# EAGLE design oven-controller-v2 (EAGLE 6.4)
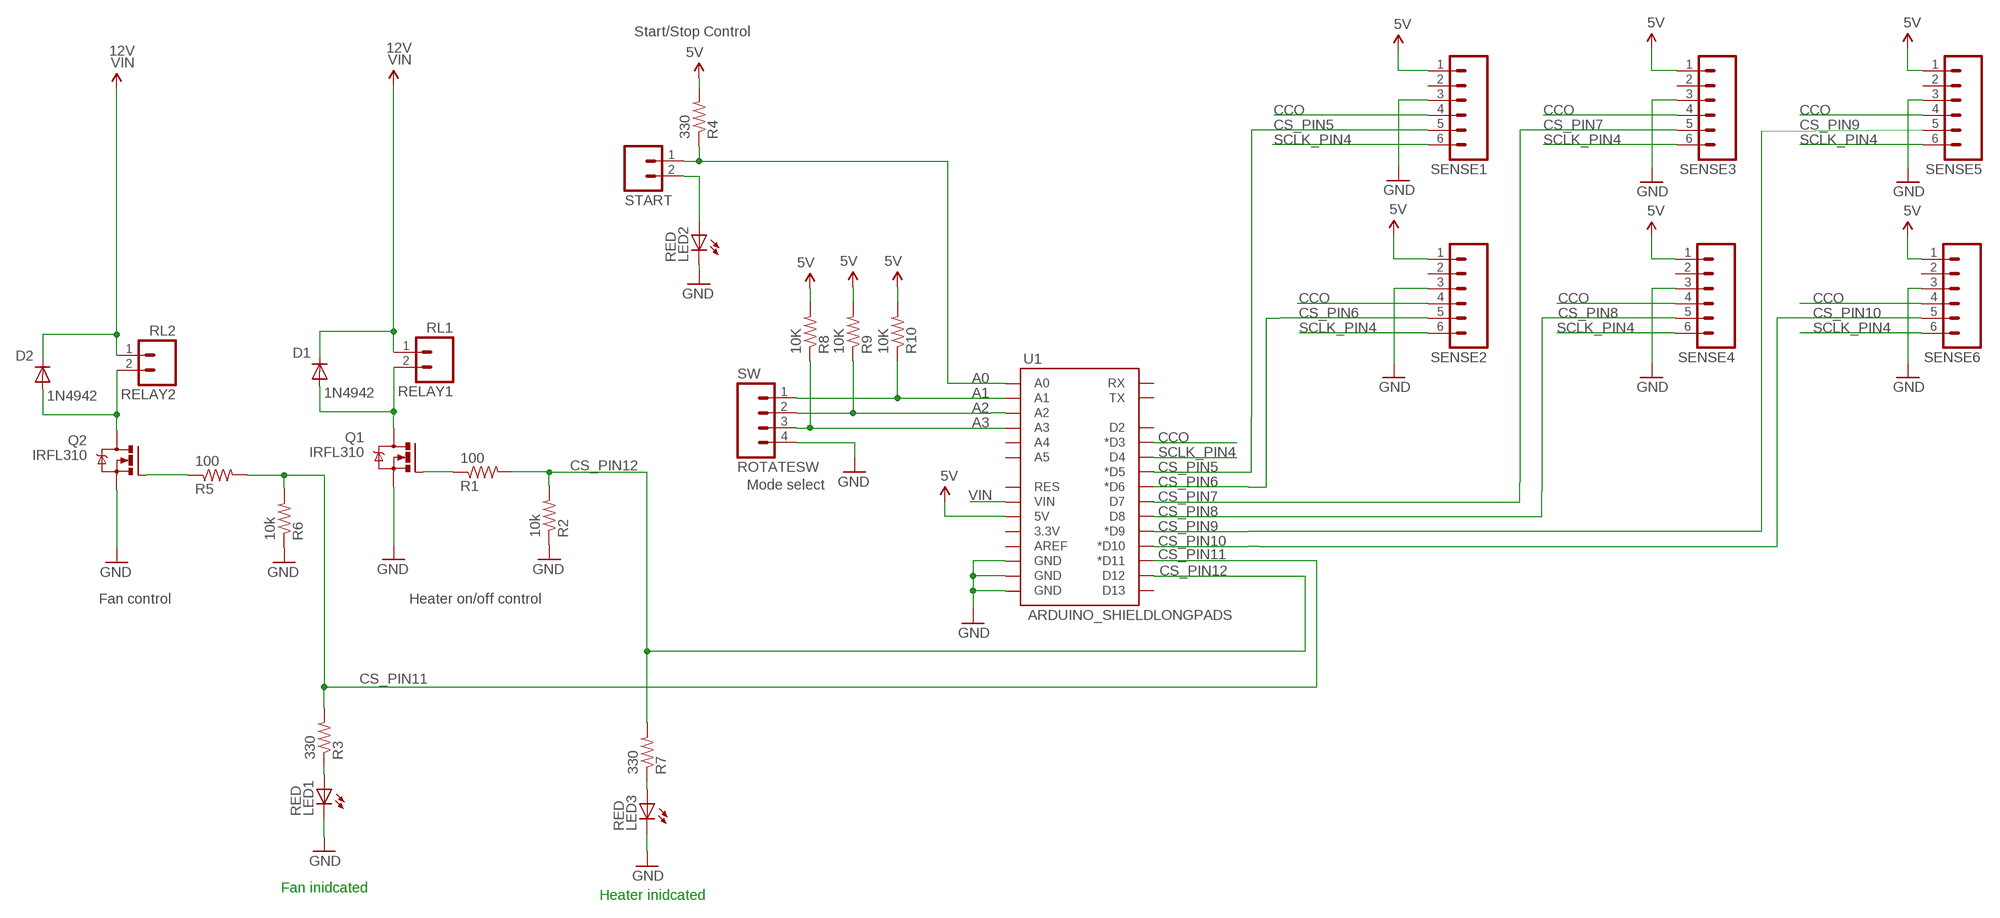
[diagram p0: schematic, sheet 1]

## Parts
D1  1N4942  [DO41-10]
D2  1N4942  [DO41-10]
LED1  RED  LED5MM  [LED5MM]
LED2  RED  LED5MM  [LED5MM]
LED3  RED  LED5MM  [LED5MM]
Q1  IRFL310  IRF520  [TO220BV]
Q2  IRFL310  IRF520  [TO220BV]
R1  100  RESISTORAXIAL-0.3  [AXIAL-0.3]
R2  10k  RESISTORAXIAL-0.3  [AXIAL-0.3]
R3  330  RESISTORAXIAL-0.3  [AXIAL-0.3]
R4  330  RESISTORAXIAL-0.3  [AXIAL-0.3]
R5  100  RESISTORAXIAL-0.3  [AXIAL-0.3]
R6  10k  RESISTORAXIAL-0.3  [AXIAL-0.3]
R7  330  RESISTORAXIAL-0.3  [AXIAL-0.3]
R8  10K  RESISTORAXIAL-0.3  [AXIAL-0.3]
R9  10K  RESISTORAXIAL-0.3  [AXIAL-0.3]
R10  10K  RESISTORAXIAL-0.3  [AXIAL-0.3]
RELAY1  RL1  M023.5MM_LOCK  [SCREWTERMINAL-3.5MM-2_LOCK]
RELAY2  RL2  M023.5MM_LOCK  [SCREWTERMINAL-3.5MM-2_LOCK]
ROTATESW  SW  M04LOCK_LONGPADS  [1X04_LOCK_LONGPADS]
SENSE1  M06LOCK_LONGPADS  [1X06_LOCK_LONGPADS]
SENSE2  M06LOCK_LONGPADS  [1X06_LOCK_LONGPADS]
SENSE3  M06LOCK_LONGPADS  [1X06_LOCK_LONGPADS]
SENSE4  M06LOCK_LONGPADS  [1X06_LOCK_LONGPADS]
SENSE5  M06LOCK_LONGPADS  [1X06_LOCK_LONGPADS]
SENSE6  M06LOCK_LONGPADS  [1X06_LOCK_LONGPADS]
START  M023.5MM_LOCK  [SCREWTERMINAL-3.5MM-2_LOCK]
U1  ARDUINO_SHIELDLONGPADS  [DUEMILANOVE_SHIELD_LONGPADS]

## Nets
5V: R4.P$2 R8.P$2 R9.P$2 R10.P$2 SENSE1.1 SENSE2.1 SENSE3.1 SENSE4.1 SENSE5.1 SENSE6.1 U1.5V
A0: R4.P$1 START.1 U1.A0
A1: R10.P$1 ROTATESW.1 U1.A1
A2: R9.P$1 ROTATESW.2 U1.A2
A3: R8.P$1 ROTATESW.3 U1.A3
CCO: SENSE1.4 SENSE2.4 SENSE3.4 SENSE4.4 SENSE5.4 SENSE6.4 U1.D3(*D3)
CS_PIN5: SENSE1.5 U1.D5(*D5)
CS_PIN6: SENSE2.5 U1.D6(*D6)
CS_PIN7: SENSE3.5 U1.D7
CS_PIN8: SENSE4.5 U1.D8
CS_PIN9: SENSE5.5 U1.D9(*D9)
CS_PIN10: SENSE6.5 U1.D10(*D10)
CS_PIN11: R3.P$2 R5.P$2 R6.P$2 U1.D11(*D11)
CS_PIN12: R1.P$2 R2.P$2 R7.P$2 U1.D12
GND: LED1.K(C) LED2.K(C) LED3.K(C) Q1.S Q2.S R2.P$1 R6.P$1 ROTATESW.4 SENSE1.3 SENSE2.3 SENSE3.3 SENSE4.3 SENSE5.3 SENSE6.3 U1.GND@0(GND) U1.GND@1(GND) U1.GND@2(GND)
N$1: Q2.G R5.P$1
N$2: Q1.G R1.P$1
N$3: D1.A Q1.D RELAY1.2
N$4: D2.A Q2.D RELAY2.2
N$7: LED1.A R3.P$1
N$9: LED3.A R7.P$1
N$10: LED2.A START.2
SCLK_PIN4: SENSE1.6 SENSE2.6 SENSE3.6 SENSE4.6 SENSE5.6 SENSE6.6 U1.D4
VIN: D1.C D2.C RELAY1.1 RELAY2.1 U1.VIN
Unconnected: SENSE1.2 SENSE2.2 SENSE3.2 SENSE4.2 SENSE5.2 SENSE6.2 U1.3.3V U1.A4 U1.A5 U1.AREF U1.D2 U1.D13 U1.RES U1.RX U1.TX

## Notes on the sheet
- Start/Stop Control
- 12V | 12V
- Mode select
- Fan control | Heater on/off control
- Fan inidcated
- Heater inidcated

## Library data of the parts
D1 D2 = diode:1N4942: DIODE
LED1-LED3 = led:LED: LED
Q1 Q2 = transistor-power:IRF520: HEXFET Power MOSFET
R1-R10 = SparkFun-Passives:RESISTOR: Resistor
RELAY1 RELAY2 START = SparkFun-Connectors:M02: Header 2
ROTATESW = SparkFun-Connectors:M04: Header 4 Standard 4-pin 0.1" header. Use with straight break away headers (SKU : PRT-00116), right angle break away headers (PRT-00553), swiss pins (PRT-00743), machine pins (PRT-00117), and female headers (PRT-00115). Molex polarized connector foot print use with SKU : PRT-08231 with associated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
SENSE1-SENSE6 = SparkFun-Connectors:M06: Header 6 Standard 6-pin 0.1" header. Use with straight break away headers (SKU : PRT-00116), right angle break away headers (PRT-00553), swiss pins (PRT-00743), machine pins (PRT-00117), and female headers (PRT-00115). Molex polarized connector foot print use with SKU : PRT-08094 with associated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
U1 = SparkFun-Boards:ARDUINO_SHIELD: Arduino shield footprint

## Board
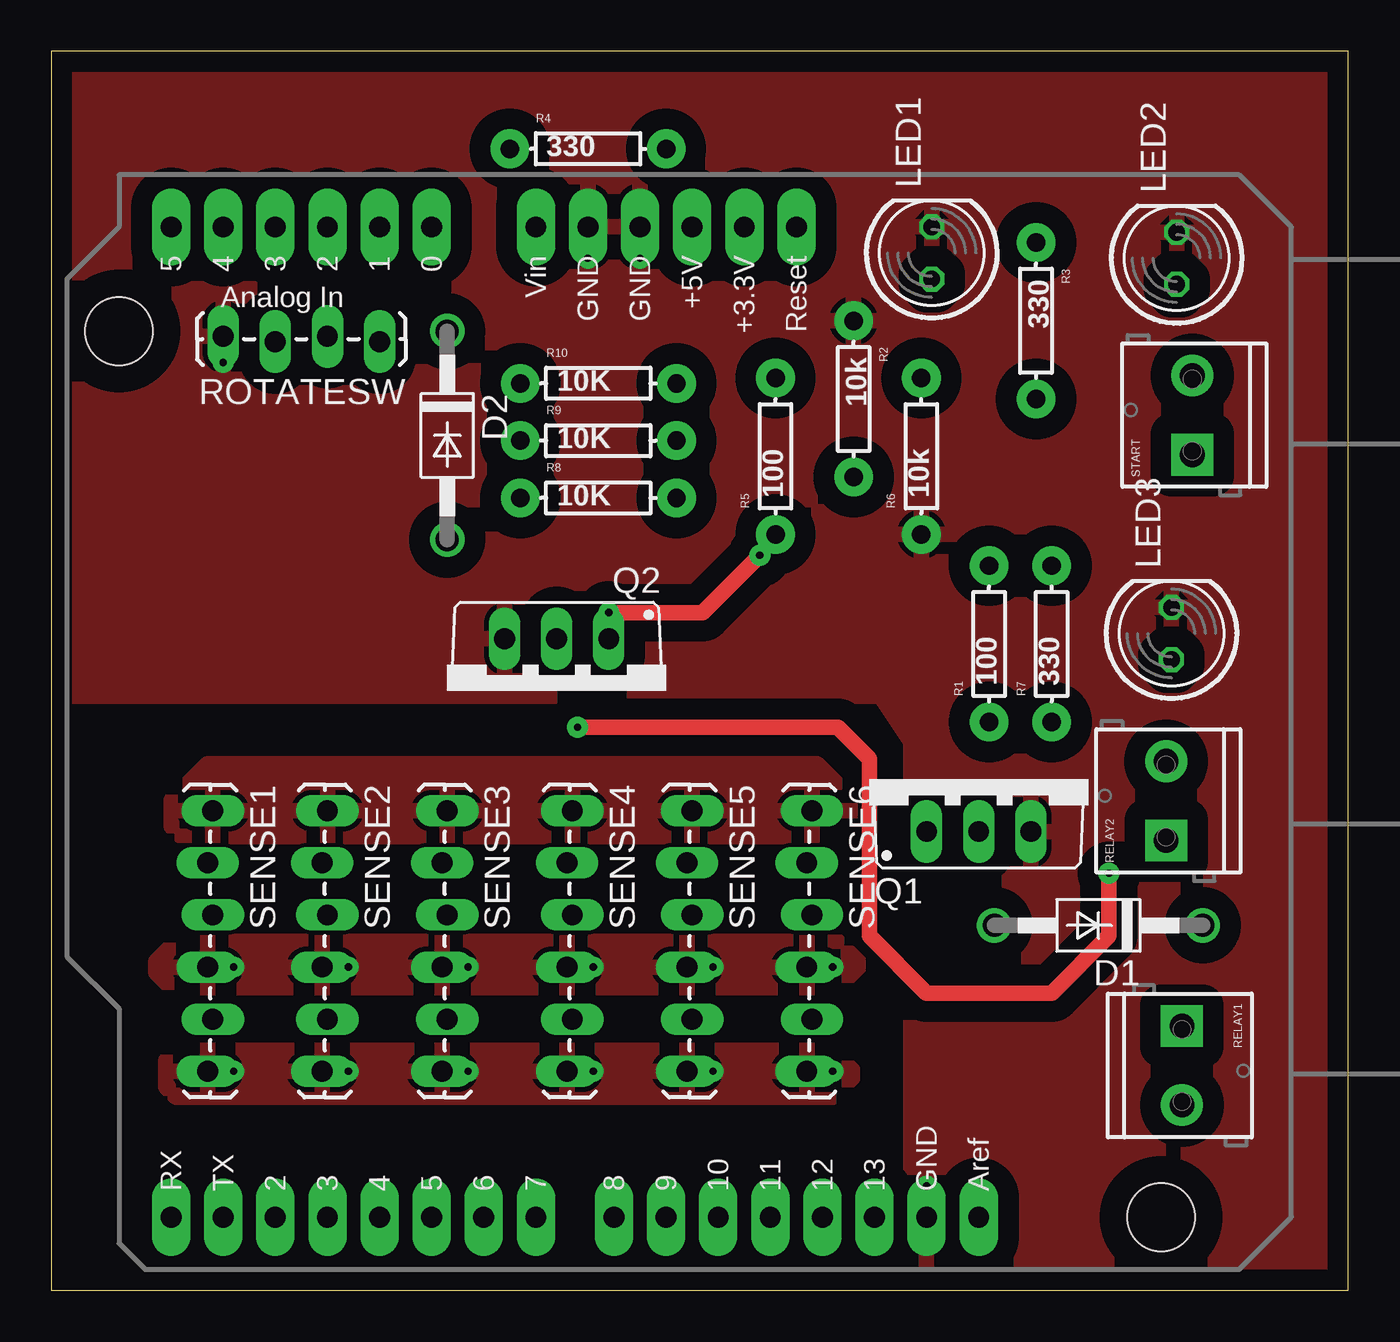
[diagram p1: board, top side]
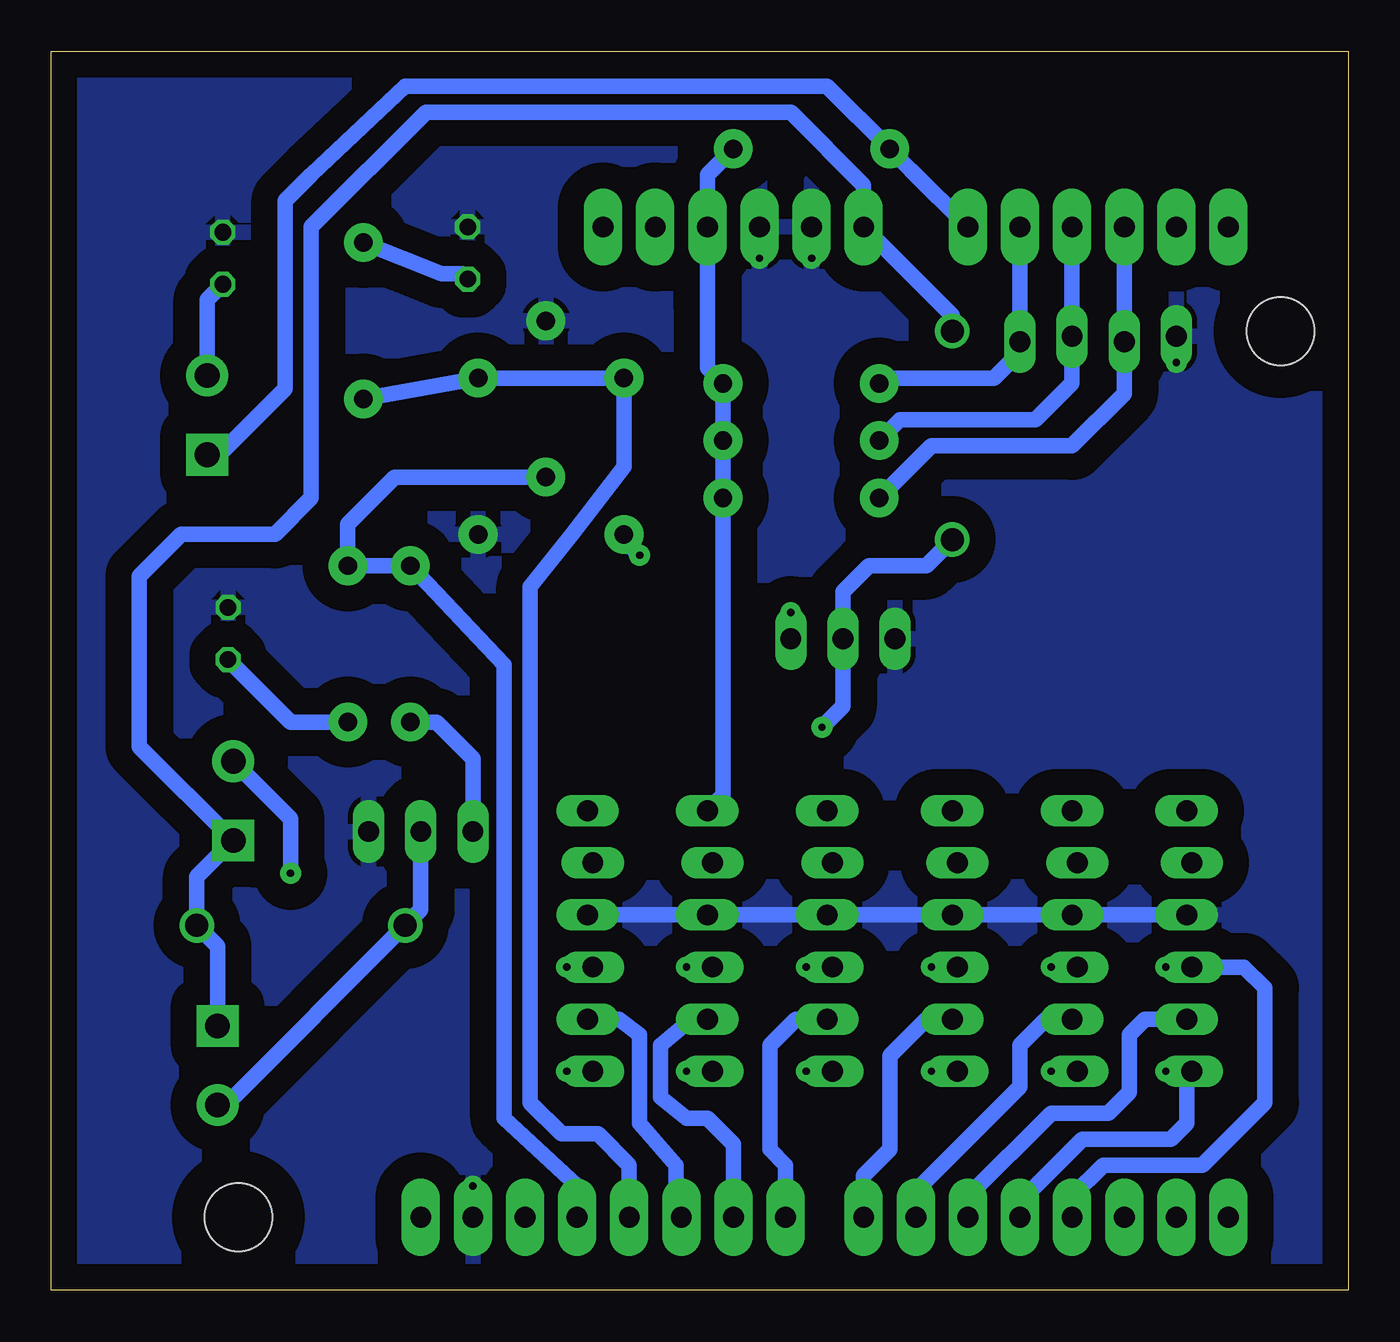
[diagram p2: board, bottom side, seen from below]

Size 63.23 x 60.38 mm. Coordinates in mm from the lower left corner, seen from the top.
Outline: 0,0 63.23,0 63.23,60.38 0,60.38 0,0
Copper layers (1*16): Top 0.0178mm / dielectric 59mil / Bottom 0.0178mm
Design rules "epl-lpkf": minimum track width 8mil, minimum drill 0.35mm, track to track 8mil, track to pad 8mil, pad to pad 8mil, via to via 8mil, smd to smd 8mil, copper to edge 15mil, drill to drill 15mil, minimum pad ring 8mil, minimum via ring 8mil, stop-mask expansion 3mil, vias tented up to drill 0mil, thermal gap 10mil

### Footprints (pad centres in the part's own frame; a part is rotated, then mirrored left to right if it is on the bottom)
DO41-10 = drill 1.118: A 5.08,0; C -5.08,0
LED5MM = drill 0.813 octagon: A -1.27,0; K 1.27,0
TO220BV = drill 1.016 long: D 0,-2.54; G -2.54,-2.54; S 2.54,-2.54
AXIAL-0.3 = drill 0.9 pad 1.88: P$1 -3.81,0; P$2 3.81,0
SCREWTERMINAL-3.5MM-2_LOCK = drill 1.2 pad 2.032 square: 1 -0.178,0 | drill 1.2 pad 2.032: 2 3.678,0
1X04_LOCK_LONGPADS = drill 1.016 long: 1 0,0; 2 2.54,-0.254; 3 5.08,0; 4 7.62,-0.254
1X06_LOCK_LONGPADS = drill 1.016 long: 1 0,0; 2 2.54,-0.254; 3 5.08,0; 4 7.62,-0.254; 5 10.16,0; 6 12.7,-0.254
DUEMILANOVE_SHIELD_LONGPADS = drill 1.016 pad 1.88 long: 3.3V 50.8,26.67; 5V 50.8,29.21; A0 50.8,41.91; A1 50.8,44.45; A2 50.8,46.99; A3 50.8,49.53; A4 50.8,52.07; A5 50.8,54.61; AREF 2.54,15.24; D2 2.54,49.53; D3 2.54,46.99; D4 2.54,44.45; D5 2.54,41.91; D6 2.54,39.37; D7 2.54,36.83; D8 2.54,33.02; D9 2.54,30.48; D10 2.54,27.94; D11 2.54,25.4; D12 2.54,22.86; D13 2.54,20.32; GND@0 50.8,31.75; GND@1 50.8,34.29; GND@2 2.54,17.78; RES 50.8,24.13; RX 2.54,54.61; TX 2.54,52.07; VIN 50.8,36.83 | hole 3.302: 45.72,57.15; 2.54,6.35

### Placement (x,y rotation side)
D1  51.05,17.78 180 top
D2  19.3,41.66 270 top
LED1  42.93,50.55 90 top
LED2  54.86,50.29 90 top
LED3  54.61,32 90 top
Q1  45.21,24.89 0 top
Q2  24.64,29.21 180 top
R1  45.72,31.5 90 top
R2  39.12,43.43 270 top
R3  48.01,47.24 270 top
R4  26.16,55.63 0 top
R5  35.31,40.64 90 top
R6  42.42,40.64 90 top
R7  48.77,31.5 90 top
R8  26.67,38.61 0 top
R9  26.67,41.4 0 top
R10  26.67,44.2 0 top
RELAY1  55.12,12.7 270 top
RELAY2  54.36,22.1 90 top
ROTATESW  16,46.23 180 top
SENSE1  7.87,23.37 270 top
SENSE2  13.46,23.37 270 top
SENSE3  19.3,23.37 270 top
SENSE4  25.4,23.37 270 top
SENSE5  31.24,23.37 270 top
SENSE6  37.08,23.37 270 top
START  55.63,40.89 90 top
U1  60.45,1.02 90 top

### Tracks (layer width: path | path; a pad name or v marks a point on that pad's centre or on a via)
5V
  Bottom 0.762: SENSE5.1 30.48,24.13 R8.P$2 R9.P$2 R10.P$2 31.24,44.96 31.24,48.01 U1.5V 31.24,54.36 R4.P$2
  pour Top: 5.84,23.88 6.6,24.64 7.62,25.65 37.34,25.65 39.12,23.88 39.12,23.11 38.1,22.1 6.35,22.1 5.84,22.61
A0
  Bottom 0.762: 18.54,51.56 U1.A0 21.34,54.61 R4.P$1 25.4,58.67 45.97,58.67 50.55,54.36 51.82,53.09 51.82,43.94 55.04,40.72 START.1
A1
  Bottom 0.762: U1.A1 ROTATESW.1 16,45.72 17.27,44.45 22.61,44.45 R10.P$1
A2
  Bottom 0.762: U1.A2 ROTATESW.2 13.46,44.2 15.24,42.42 21.84,42.42 R9.P$1
A3
  Bottom 0.762: U1.A3 ROTATESW.3 10.92,43.69 13.46,41.15 20.32,41.15 R8.P$1
CCO  (via drill 0.36 pad 1.02)
  Bottom 0.762: U1.D3 13.46,4.57 11.94,6.1 7.11,6.1 4.06,9.14 4.06,14.73 5.08,15.75 SENSE1.4
  other vias: 8.89,15.75 14.48,15.75 20.32,15.75 26.42,15.75 32.26,15.75 38.1,15.75
  pour Top: 6.6,16.76 5.84,16.76 5.08,16 5.08,15.49 5.84,14.73 38.35,14.73 39.37,15.75 39.37,16 38.35,17.02 6.86,17.02
CS_PIN5
  Bottom 0.762: SENSE1.5 9.91,13.21 10.67,12.45 10.67,9.65 11.43,8.89 11.68,8.64 14.48,8.64 18.54,4.57 U1.D5
CS_PIN6
  Bottom 0.762: SENSE2.5 14.73,13.21 16,11.94 16,9.91 20.83,5.08 21.08,4.83 U1.D6
CS_PIN7
  Bottom 0.762: SENSE3.5 20.57,13.21 22.35,11.43 22.35,6.86 23.62,5.59 U1.D7
CS_PIN8
  Bottom 0.762: SENSE4.5 26.92,13.21 28.19,11.94 28.19,6.86 27.43,6.1 U1.D8
CS_PIN9
  Bottom 0.762: SENSE5.5 32,13.21 33.53,11.94 33.53,9.4 32.26,8.38 31.24,8.38 29.97,7.11 U1.D9
CS_PIN10
  Bottom 0.762: SENSE6.5 35.56,13.21 34.54,12.45 34.54,8.13 32.77,6.1 32.77,3.81 U1.D10
CS_PIN11
  Bottom 0.762: R3.P$2 R6.P$2 R5.P$2 35.31,40.13 37.85,36.83 39.88,34.29 39.88,9.14 38.35,7.62 36.58,7.62 35.05,6.1 U1.D11
CS_PIN12
  Bottom 0.762: R2.P$2 46.48,39.62 48.77,37.34 R7.P$2 R1.P$2 41.15,30.48 41.15,8.38 37.59,5.08 U1.D12
GND  (via drill 0.36 pad 1.02)
  Bottom 0.762: SENSE1.3 SENSE2.3 SENSE3.3 SENSE4.3 SENSE5.3 SENSE6.3
  other vias: 28.7,50.29 26.16,50.29 8.38,45.21 42.67,5.08
  pour Bottom (isolate 1.27): -1.27,56.9 -1.27,-1.27 65.02,-1.27 64.52,61.47 -1.52,61.47
  pour Top (isolate 1.016): -1.52,61.72 -1.02,28.96 40.39,28.96 41.91,26.67 41.91,-0.25 65.02,-0.51 65.53,2.29 65.28,28.96 64.77,61.72
N$1  (via drill 0.36 pad 1.02)
  Top 0.762: v27.18,33.02 31.75,33.02 v34.54,35.81
  Bottom 0.762: Q2.G v27.18,33.02 | R5.P$1 35.31,36.58 v34.54,35.81
N$2
  Bottom 0.762: R1.P$1 44.45,27.69 42.67,25.91 Q1.G
N$3
  Bottom 0.762: RELAY1.2 54.73,9.02 D1.A 45.21,18.54 Q1.D
N$4  (via drill 0.36 pad 1.02)
  Top 0.762: v25.65,27.43 38.35,27.43 39.88,25.91 39.88,17.27 42.67,14.48 48.77,14.48 51.56,17.27 v51.56,20.32
  Bottom 0.762: D2.A 20.57,35.31 23.37,35.31 24.64,34.04 Q2.D 24.64,28.45 v25.65,27.43 | v51.56,20.32 51.56,22.98 RELAY2.2
N$7
  Bottom 0.762: R3.P$1 44.2,49.53 43.18,49.53 LED1.A
N$9
  Bottom 0.762: R7.P$1 51.56,27.69 LED3.A
N$10
  Bottom 0.762: START.2 55.63,48.26 LED2.A
SCLK_PIN4  (via drill 0.36 pad 1.02)
  Bottom 0.762: U1.D4 16,4.32 12.95,7.37 8.64,7.37 7.87,8.13 7.87,10.41 SENSE1.6
  other vias: 8.89,10.67 14.48,10.67 20.32,10.67 26.42,10.67 32.26,10.67 38.1,10.67
  pour Top: 38.35,11.43 39.12,10.67 39.12,10.41 38.1,9.4 6.1,9.4 5.59,9.91 5.59,11.18 6.1,11.68 37.85,11.68 38.35,11.18
VIN
  Bottom 0.762: RELAY1.1 55.12,16.76 D1.C 56.13,20.14 RELAY2.1 58.93,26.49 58.93,34.8 56.9,36.83 52.32,36.83 50.55,38.61 50.55,51.82 44.96,57.4 27.18,57.4 23.62,53.85 U1.VIN 19.3,47.5 D2.C

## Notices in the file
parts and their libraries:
SparkFun-Boards: Licensing: CC v3.0 Share-Alike You are welcome to use this library for commercial purposes.
